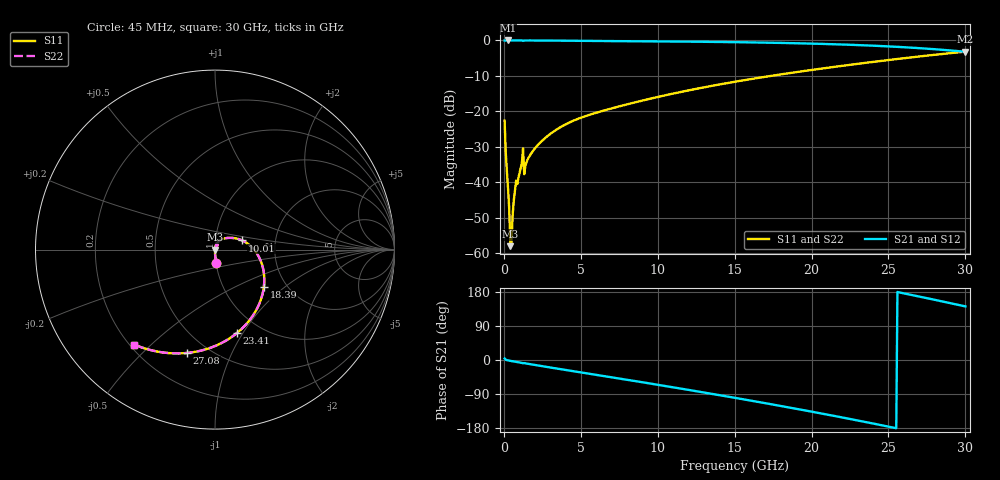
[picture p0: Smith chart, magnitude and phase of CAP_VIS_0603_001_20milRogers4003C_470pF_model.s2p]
! S-parameter model data by Modelithics Inc.  support@modelithics.com  813-866-6335  Tampa FL USA
! S-Parameter data specifications:
! Substrate: 20-mil Rogers 4003C, substrate thickness, H=0.508mm, Dielectric constant, Er=3.75
! PCB Mounting Pad Footprint: Pad width, PadW=0.90mm , Pad length, PadL=1.00mm , Pad gap, PadG (edge-to-edge)=1.00mm , Reference planes=3.0mm apart
! Created Wed Nov 18 13:35:11 2015
# hz S ma R 50
! 2 Port Network Data from SP1.SP block
! freq  magS11  angS11  magS21  angS21  magS12  angS12  magS22  angS22
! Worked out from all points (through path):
!   401 points, 45 MHz to 30 GHz, reference 50 ohm
!   highest |S21| = 0.00 dB at 269.7 MHz (marker M1); lowest = -3.2 dB at 30 GHz (marker M2)
!   group delay of S21, straight-line fit = 20 ps
!   lowest |S11| = -58.0 dB at 419.4 MHz (marker M3), VSWR 1.00, Z = 50 - j0.12 ohm
!   |S11| at or under -10 dB: start of sweep to 17.34 GHz
!   |S22| runs from -58.0 to -3.2 dB; largest |S21 - S12| = 0
!   S11 on the Smith chart (normalised r, x): 45 MHz: 1.00, -0.15; 10.01 GHz: 1.35, +0.14; 18.39 GHz: 1.54, -0.72; 23.41 GHz: 0.78, -0.94; 27.08 GHz: 0.38, -0.69; 30 GHz: 0.22, -0.44
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4.5e7  0.07416 -85.9  0.9971 4.0  0.9971 4.0  0.07416 -85.9
1.94775e8  0.01419 -89.0  0.9996 -0.3  0.9996 -0.3  0.01419 -89.0
2.696625e8  0.008149 -88.6  0.9996 -1.1  0.9996 -1.1  0.008149 -88.6
3.4455e8  0.004203 -86.3  0.9996 -1.7  0.9996 -1.7  0.004203 -86.3
4.194375e8  0.001263 -72.5  0.9995 -2.3  0.9995 -2.3  0.001263 -72.5
5.692125e8  0.003543 78.4  0.9994 -3.4  0.9994 -3.4  0.003543 78.4
7.189875e8  0.007813 80.3  0.9992 -4.5  0.9992 -4.5  0.007813 80.3
1.093425e9  0.01566 79.8  0.9989 -7.1  0.9989 -7.1  0.01566 79.8
1.467862e9  0.01921 77.8  0.9988 -9.4  0.9988 -9.4  0.01921 77.8
1.917188e9  0.02829 75.3  0.9983 -12.4  0.9983 -12.4  0.02829 75.3
2.890725e9  0.04597 68.0  0.9962 -18.9  0.9962 -18.9  0.04597 68.0
5.062462e9  0.08232 49.5  0.9857 -33.2  0.9857 -33.2  0.08232 49.5
1.000504e10  0.1599 18.6  0.9696 -65.4  0.9696 -65.4  0.1599 18.6
1.007992e10  0.1612 18.1  0.9694 -65.9  0.9694 -65.9  0.1612 18.1
1.26261e10  0.2106 2.2  0.9594 -83.2  0.9594 -83.2  0.2106 2.2
1.50225e10  0.262 -13.7  0.9462 -99.9  0.9462 -99.9  0.262 -13.7
1.839244e10  0.3422 -37.3  0.9195 -124.2  0.9195 -124.2  0.3422 -37.3
2.003996e10  0.385 -49.4  0.9021 -136.6  0.9021 -136.6  0.385 -49.4
2.34099e10  0.4806 -75.3  0.8543 -162.9  0.8543 -162.9  0.4806 -75.3
2.505742e10  0.5315 -88.5  0.8234 -176.3  0.8234 -176.3  0.5315 -88.5
2.707939e10  0.5972 -105.3  0.7771 166.8  0.7771 166.8  0.5972 -105.3
3e10  0.6949 -130.5  0.6922 141.4  0.6922 141.4  0.6949 -130.5
